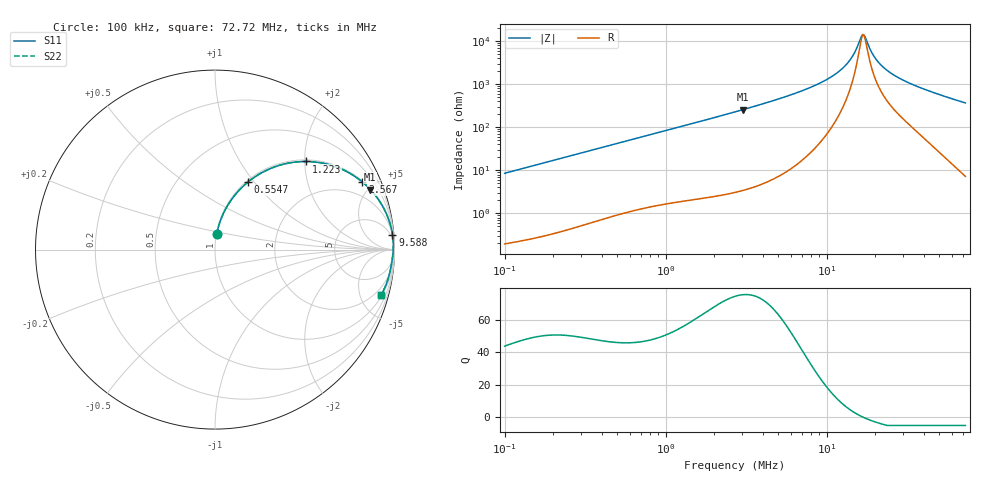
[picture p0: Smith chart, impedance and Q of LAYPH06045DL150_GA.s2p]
! LAYPH06045DL150_GA  S-PARAMETER MODEL  ( General Type )
! Model Generated by TAIYO YUDEN Corporation (http://www.ty-top.com)
! Version 2.0
! TAIYO YUDEN Control No. 180914NI43SB-FBB
! Copyright(c) 2018 TAIYO YUDEN CO.,LTD. All Rights Reserved.
! Product Description (link to TY-COMPAS)
! https://ds.yuden.co.jp/TYCOMPAS/or/detail?pn=LAYPH06045DL150MGA&u=M
! Products Name : Inductors
! Characteristics :
!  Inductance : 15 uH , SRF(min) : -Hz , DC Resistance(max) : 0.0768 Ohm
!  Rated Current : Saturation :1.7 A , Temp Rise : 1.4 A (25 degC)
!  Case Size : 6.3 x 6.0 / 0.248 x 0.236 [mm/inch] , Thickness : 4.5 / 0.177 [mm/inch]
!  (Conditions: Temperature = 25 degC , DC Bias Current/Voltage = 0A / 0V)
! External Node Assignments :
!  1  o---GGG---o  2
! GND o---------o GND
! Frequency Range : 0.1MHz  -  72.722828MHz  [ 402 STEP ]
# MHz S RI R 50
! Freq[MHz].  S11 Real  S11 Imag  S21 Real  S21 Imag  S12 Real  S12 Imag  S22 Real  S22 Imag
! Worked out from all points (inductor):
!   401 points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, 100 kHz to 72.72 MHz, reference 50 ohm
!   read as one part in series: L = 13.6 uH near 103.3 kHz
!   highest Q = 75.3 at 3.026 MHz (marker M1), where L = 13.5 uH
!   self-resonance near 16.79 MHz
!   S11 on the Smith chart (normalised r, x): 100 kHz: 1.00, +0.17; 554.7 kHz: 1.02, +0.93; 1.223 MHz: 1.04, +2.03; 2.567 MHz: 1.06, +4.33; 9.588 MHz: 2, +24; 72.72 MHz: 1.14, -7.35
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0.1  0.00914 0.0844  0.9909 -0.0844  0.9909 -0.0844  0.00914 0.0844
0.30153  0.0653 0.2371  0.9347 -0.2371  0.9347 -0.2371  0.0653 0.2371
0.55467  0.1833 0.3761  0.8167 -0.3761  0.8167 -0.3761  0.1833 0.3761
0.909201  0.3673 0.472  0.6327 -0.472  0.6327 -0.472  0.3673 0.472
1.223024  0.5084 0.4909  0.4916 -0.4909  0.4916 -0.4909  0.5084 0.4909
2.566687  0.8206 0.377  0.1794 -0.377  0.1794 -0.377  0.8206 0.377
2.741508  0.8398 0.3602  0.1602 -0.3602  0.1602 -0.3602  0.8398 0.3602
3.026318  0.8656 0.3346  0.1344 -0.3346  0.1344 -0.3346  0.8656 0.3346
5.298545  0.9562 0.1966  0.0438 -0.1966  0.0438 -0.1966  0.9562 0.1966
8.131398  0.9837 0.1116  0.0163 -0.1116  0.0163 -0.1116  0.9837 0.1116
9.587536  0.9889 0.0836  0.0111 -0.0836  0.0111 -0.0836  0.9889 0.0836
11.49219  0.9922 0.0551  0.00775 -0.0551  0.00775 -0.0551  0.9922 0.0551
13.32878  0.9935 0.0332  0.00654 -0.0332  0.00654 -0.0332  0.9935 0.0332
14.71349  0.9936 0.0191  0.00638 -0.0191  0.00638 -0.0191  0.9936 0.0191
16.24204  0.9933 0.00539  0.00669 -0.00539  0.00669 -0.00539  0.9933 0.00539
16.78607  0.9931 0.000872  0.00689 -0.000872  0.00689 -0.000872  0.9931 0.000872
17.34832  0.9929 -0.00362  0.00713 0.00362  0.00713 0.00362  0.9929 -0.00362
18.83772  0.9921 -0.0148  0.00792 0.0148  0.00792 0.0148  0.9921 -0.0148
20.12079  0.9913 -0.0236  0.00873 0.0236  0.00873 0.0236  0.9913 -0.0236
24.51857  0.988 -0.0502  0.012 0.0502  0.012 0.0502  0.988 -0.0502
37.01259  0.9777 -0.1109  0.0223 0.1109  0.0223 0.1109  0.9777 -0.1109
72.72283  0.9268 -0.2508  0.0732 0.2508  0.0732 0.2508  0.9268 -0.2508
